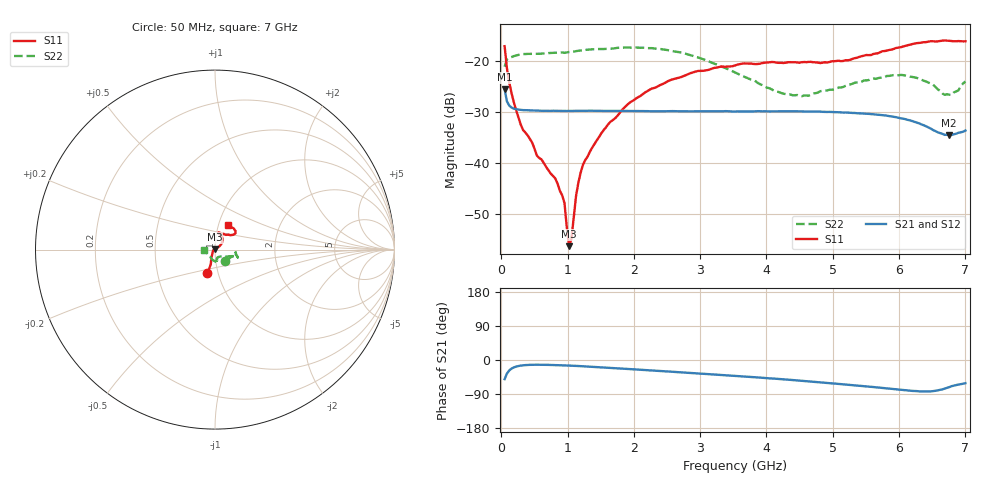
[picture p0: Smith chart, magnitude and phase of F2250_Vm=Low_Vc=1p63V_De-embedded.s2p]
! Integrated Device Technology
! Corporate Headquarters
! 6024 Silver Creek Valley Road
! San Jose, CA 95138  USA
! Phone:  1-408-284-8200
! Toll Free:  1-800-223-1366
! Webpage:  http://www.idt.com/
! Timing and RF Division
! 515 Groton Road, Suite 102
! Westford, MA 01886-6024
! Device:  F2250
! Description: Voltage Variable RF Attenuator
! Frequency:  50.0 -  6000.00 MHz
! Package:  3x3 mm Thin QFN Plastic Package: 16 pin
! Ports:  2 RF, 3 DC
!  Pin  1  = GND
!  Pin  2  = NC
!  Pin  3  = RF1  = Port 1
!  Pin  4  = NC
!  Pin  5  = GND
!  Pin  6  = GND
!  Pin  7  = GND
!  Pin  8  = GND
!  Pin  9  = NC
!  Pin 10  = RF2  = Port 2
!  Pin 11  = NC
!  Pin 12  = GND
!  Pin 13  = GND
!  Pin 14  = VCNTRL
!  Pin 15  = VDD
!  Pin 16  = VMODE
! Vcntrl:  1.630 Volts
! Vmode:  +0.000 Volts
! Vdd:  +3.30  Volts
! Current:  1.189 mA
! Data:  The device was measured on a the F2250 evaluation board which has
!  individual transmission lines to the RF pins.  Data was collected
!  using a calibrated network analyzer.  The evaluation board was
!  de-embedded using a TRL calibration technique.
!  The reference plane is the edge of the package pin.
! Misc:  SN 10
!  Action Tracker AT0258
! Date Measured:  2014-11-26
! Date:  2015-10-15  MJV
! Note:
!  Integrated Device Technology supplies this data as a sample of measured
!  data at the package pin for this product.  Your particular data for this
!  product may vary.
!  Data was taken at 25 degrees C.
!  Integrated Device Technology reserves the right to change this data at anytime.
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# GHz S dB R 50
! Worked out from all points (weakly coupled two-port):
!   201 points, 50 MHz to 7 GHz, reference 50 ohm
!   highest |S21| = -25.58 dB at 50 MHz (marker M1); lowest = -34.5 dB at 6.757 GHz (marker M2)
!   lowest |S11| = -56.2 dB at 1.023 GHz (marker M3), VSWR 1.00, Z = 49.9 + j0.126 ohm
!   |S11| at or under -10 dB: start of sweep to end of sweep
!   |S22| runs from -26.9 to -17.4 dB; largest |S21 - S12| = 0.00013
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0.05  -17.15 -107.5  -25.58 -50.6  -25.59 -50.6  -21.17 -48.1
0.1195  -24.22 -110.0  -28.76 -27.6  -28.75 -27.6  -19.43 -13.9
0.29325  -32.47 -123.9  -29.60 -14.8  -29.59 -14.8  -18.74 -8.7
0.5365  -38.52 -150.2  -29.74 -12.5  -29.77 -12.5  -18.66 -8.6
0.8145  -43.01 174.9  -29.79 -13.4  -29.79 -13.4  -18.46 -11.9
0.91875  -46.32 156.9  -29.81 -14.1  -29.78 -14.1  -18.38 -13.5
0.9535  -47.81 173.5  -29.82 -14.3  -29.81 -14.3  -18.46 -13.6
1.023  -56.23 125.1  -29.82 -14.8  -29.80 -14.8  -18.30 -13.8
1.05775  -54.85 87.4  -29.83 -15.0  -29.80 -15.0  -18.26 -14.0
1.12725  -46.45 44.3  -29.80 -15.6  -29.80 -15.6  -18.13 -14.9
1.2315  -40.36 34.5  -29.78 -16.5  -29.77 -16.6  -17.94 -16.3
1.6485  -31.91 38.2  -29.82 -20.8  -29.81 -20.8  -17.66 -17.6
1.9265  -28.30 38.9  -29.82 -23.9  -29.83 -23.9  -17.44 -18.3
2.37825  -24.87 45.7  -29.88 -28.8  -29.85 -28.8  -17.67 -18.7
2.93425  -22.11 58.8  -29.88 -35.0  -29.87 -35.1  -19.20 -19.9
3.525  -20.92 71.7  -29.93 -41.9  -29.91 -41.9  -22.30 -30.4
4.25475  -20.44 77.4  -29.88 -50.9  -29.90 -50.9  -26.44 -55.0
4.7065  -20.30 71.9  -29.93 -57.4  -29.93 -57.4  -26.40 -73.0
5.85325  -17.89 40.0  -30.83 -75.8  -30.80 -75.8  -22.96 -79.5
6.305  -16.52 40.2  -32.25 -82.7  -32.26 -82.7  -23.50 -88.8
6.75675  -16.11 50.8  -34.52 -71.6  -34.56 -71.5  -26.65 -141.7
7  -16.20 62.9  -33.64 -61.3  -33.59 -61.4  -24.04 179.7
